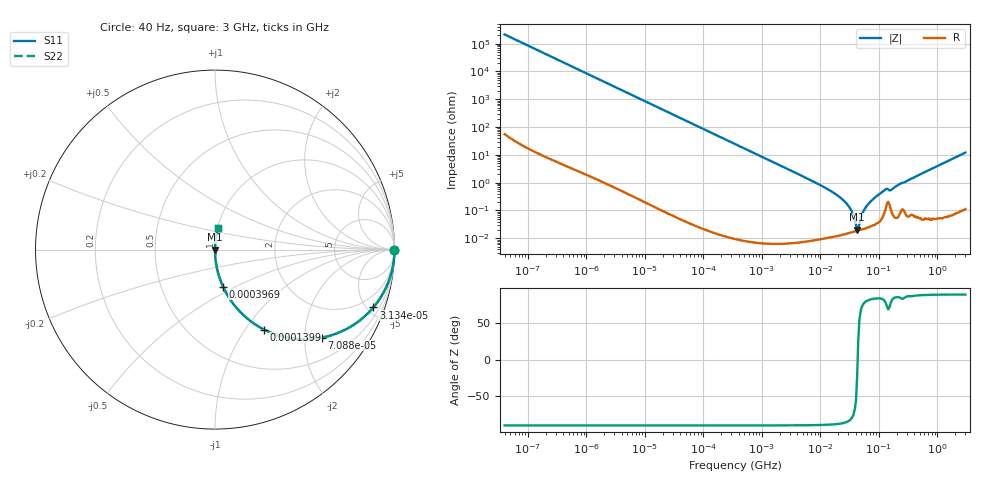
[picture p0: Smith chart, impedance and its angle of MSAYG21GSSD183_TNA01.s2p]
! MSAYG21GSSD183_TNA01  S-PARAMETER MODEL  ( General Type )
! Model Generated by TAIYO YUDEN Corporation (http://www.ty-top.com)
! Version 2.0
! TAIYO YUDEN Control No. 031016
! Copyright(c) 2003 TAIYO YUDEN CO.,LTD. All Rights Reserved.
! Product Description (link to TY-COMPAS)
! https://ds.yuden.co.jp/TYCOMPAS/or/detail?pn=MSAYG21GSSD183KTNA01&u=M
! Products Name : Multilayer Ceramic Capacitors
! Characteristics :
!  Capacitance : 0.018 uF , Rated Voltage : 35V
!  Case Size : 2.0 x 1.25 / 0.079 x 0.049 [mm/inch] , Thickness : 1.25 / 0.049 [mm/inch]
!  (Conditions: Temperature = 25 degC , DC Bias Current/Voltage = 0A / 0V)
! External Node Assignments :
!  1  o---| |---o  2
! GND o---------o GND
! Frequency Range : 40Hz  -  3GHz  [ 401 STEP ]
# MHz S RI R 50
! Freq[MHz].  S11 Real  S11 Imag  S21 Real  S21 Imag  S12 Real  S12 Imag  S22 Real  S22 Imag
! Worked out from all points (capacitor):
!   401 points, 40 Hz to 3 GHz, reference 50 ohm
!   read as one part in series: C = 18.5 nF near 44 Hz
!   lowest |Z| = 20.2 mohm at 42.31 MHz (marker M1)
!   series resonance near 43.22 MHz, so ESL is about 730 pH
!   S11 on the Smith chart (normalised r, x): 40 Hz: open; 31.34 kHz: 1.00, -5.48; 70.88 kHz: 1.00, -2.42; 139.9 kHz: 1.00, -1.23; 396.9 kHz: 1.00, -0.43; 3 GHz: 1.00, +0.24
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4e-05  1 -0.000466  3.38e-07 0.000466  3.38e-07 0.000466  1 -0.000466
0.000834  0.9999 -0.00972  9.66e-05 0.00972  9.66e-05 0.00972  0.9999 -0.00972
0.00535  0.9961 -0.0621  0.00389 0.0621  0.00389 0.0621  0.9961 -0.0621
0.017386  0.9605 -0.1946  0.0395 0.1946  0.0395 0.1946  0.9605 -0.1946
0.031343  0.8823 -0.3222  0.1177 0.3222  0.1177 0.3222  0.8823 -0.3222
0.07088  0.5944 -0.4909  0.4056 0.4909  0.4056 0.4909  0.5944 -0.4909
0.139906  0.2734 -0.4456  0.7266 0.4456  0.7266 0.4456  0.2734 -0.4456
0.362475  0.0531 -0.2241  0.9469 0.2241  0.9469 0.2241  0.0531 -0.2241
0.396875  0.0447 -0.2065  0.9553 0.2065  0.9553 0.2065  0.0447 -0.2065
1.28983  0.00446 -0.0662  0.9955 0.0662  0.9955 0.0662  0.00446 -0.0662
7.222098  0.000215 -0.0115  0.9998 0.0115  0.9998 0.0115  0.000215 -0.0115
15.60822  0.000132 -0.00476  0.9999 0.00476  0.9999 0.00476  0.000132 -0.00476
25.69909  0.000143 -0.00214  0.9999 0.00214  0.9999 0.00214  0.000143 -0.00214
32.2371  0.000159 -0.00117  0.9998 0.00117  0.9998 0.00117  0.000159 -0.00117
40.43842  0.00018 -0.000268  0.9998 0.000268  0.9998 0.000268  0.00018 -0.000268
42.31378  0.000185 -8.2e-05  0.9998 8.2e-05  0.9998 8.2e-05  0.000185 -8.2e-05
46.32945  0.000195 0.000281  0.9998 -0.000281  0.9998 -0.000281  0.000195 0.000281
55.54024  0.000219 0.001  0.9998 -0.001  0.9998 -0.001  0.000219 0.001
69.67004  0.000259 0.00195  0.9997 -0.00195  0.9997 -0.00195  0.000259 0.00195
125.5988  0.000917 0.00539  0.9991 -0.00539  0.9991 -0.00539  0.000917 0.00539
150.5692  0.00168 0.00501  0.9983 -0.00501  0.9983 -0.00501  0.00168 0.00501
3000  0.0154 0.1186  0.9846 -0.1186  0.9846 -0.1186  0.0154 0.1186
